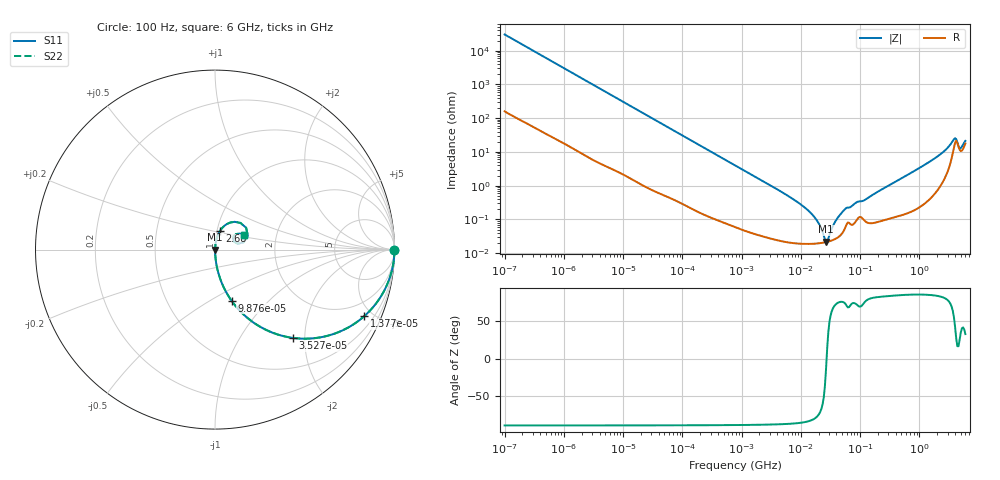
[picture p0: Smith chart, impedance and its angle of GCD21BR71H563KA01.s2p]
!Murata Part Number: GCD21BR71H563KA01
!These Parameters are Measured in Series Mode Connection
!Data Generated on Mar 13, 2026
!  o--ll--o
!Port1  Port2
!  o------o
!Operation Temp=25[degC], DC Bias Voltage=0[V]
!Freq. Start=100[Hz] Stop=6[GHz] 401[Steps]
# Hz S RI R 50
!Freq.(Hz) S11(Real) S11(Imag) S21(Real) S21(Imag) S12(Real) S12(Imag) S22(Real) S22(Imag)
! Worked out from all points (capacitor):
!   401 points, 100 Hz to 6 GHz, reference 50 ohm
!   read as one part in series: C = 52.7 nF near 109 Hz
!   lowest |Z| = 21.9 mohm at 26.62 MHz (marker M1)
!   series resonance near 27.26 MHz, so ESL is about 650 pH
!   S11 on the Smith chart (normalised r, x): 100 Hz: open; 13.77 kHz: 1.03, -4.46; 35.27 kHz: 1.01, -1.75; 98.76 kHz: 1.01, -0.63; 2.68 GHz: 1.03, +0.21; 6 GHz: 1.36, +0.23
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100  1 -0.00331  2.85e-05 0.00331  2.85e-05 0.00331  1 -0.00331
2008  0.9953 -0.0655  0.0047 0.0655  0.0047 0.0655  0.9953 -0.0655
6728  0.9527 -0.2089  0.0473 0.2089  0.0473 0.2089  0.9527 -0.2089
13772  0.8311 -0.3712  0.1689 0.3712  0.1689 0.3712  0.8311 -0.3712
35265  0.4341 -0.4919  0.5659 0.4919  0.5659 0.4919  0.4341 -0.4919
40335  0.3704 -0.479  0.6296 0.479  0.6296 0.479  0.3704 -0.479
98762  0.092 -0.2844  0.908 0.2844  0.908 0.2844  0.092 -0.2844
252896  0.0162 -0.1212  0.9838 0.1212  0.9838 0.1212  0.0162 -0.1212
774597  0.00223 -0.0404  0.9978 0.0404  0.9978 0.0404  0.00223 -0.0404
6644369  0.000224 -0.00452  0.9998 0.00452  0.9998 0.00452  0.000224 -0.00452
1.555665e7  0.000191 -0.00139  0.9998 0.00139  0.9998 0.00139  0.000191 -0.00139
1.946e7  0.000195 -0.000809  0.9998 0.000809  0.9998 0.000809  0.000195 -0.000809
2.662322e7  0.000212 -5.54e-05  0.9998 5.54e-05  0.9998 5.54e-05  0.000212 -5.54e-05
2.911731e7  0.000221 0.000157  0.9998 -0.000157  0.9998 -0.000157  0.000221 0.000157
3.983537e7  0.000275 0.000937  0.9997 -0.000937  0.9997 -0.000937  0.000275 0.000937
5.449875e7  0.000506 0.00187  0.9995 -0.00187  0.9995 -0.00187  0.000506 0.00187
3.124326e8  0.00116 0.0103  0.9988 -0.0103  0.9988 -0.0103  0.00116 0.0103
1.309207e9  0.00513 0.0439  0.9949 -0.0439  0.9949 -0.0439  0.00513 0.0439
2.679998e9  0.0269 0.1027  0.9731 -0.1027  0.9731 -0.1027  0.0269 0.1027
3.8344e9  0.1417 0.1487  0.8583 -0.1487  0.8583 -0.1487  0.1417 0.1487
5.016141e9  0.0999 0.0608  0.9001 -0.0608  0.9001 -0.0608  0.0999 0.0608
6e9  0.1593 0.0824  0.8407 -0.0824  0.8407 -0.0824  0.1593 0.0824
